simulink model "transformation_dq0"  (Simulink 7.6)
settings: Solver=ode45  StartTime=0.0  StopTime=10.0  RelTol=1e-3
libraries: powerlib_extras x3

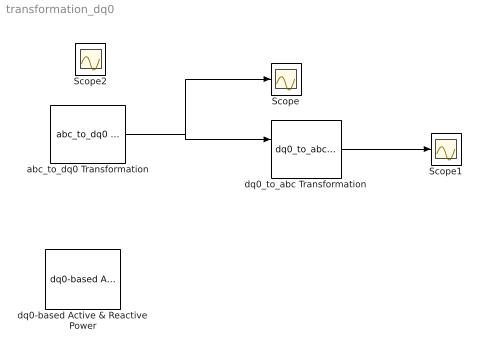
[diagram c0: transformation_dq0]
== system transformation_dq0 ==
  Scope : Scope
  Scope1 : Scope
  Scope2 : Scope
  abc_to_dq0 Transformation : powerlib_extras/Measurements/abc_to_dq0 Transformation  DialogController=POWERSYS.PowerSysDialog  SystemSampleTime=-1
  dq0-based Active & Reactive Power : powerlib_extras/Measurements/dq0-based Active & Reactive Power  DialogController=POWERSYS.PowerSysDialog  SystemSampleTime=-1
  dq0_to_abc Transformation : powerlib_extras/Measurements/dq0_to_abc Transformation  DialogController=POWERSYS.PowerSysDialog  SystemSampleTime=-1
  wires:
  abc_to_dq0 Transformation/1 -> dq0_to_abc Transformation/1, Scope/1
  ? -> abc_to_dq0 Transformation/2, dq0_to_abc Transformation/2
  dq0_to_abc Transformation/1 -> Scope1/1
  ? -> abc_to_dq0 Transformation/1, Scope2/1
